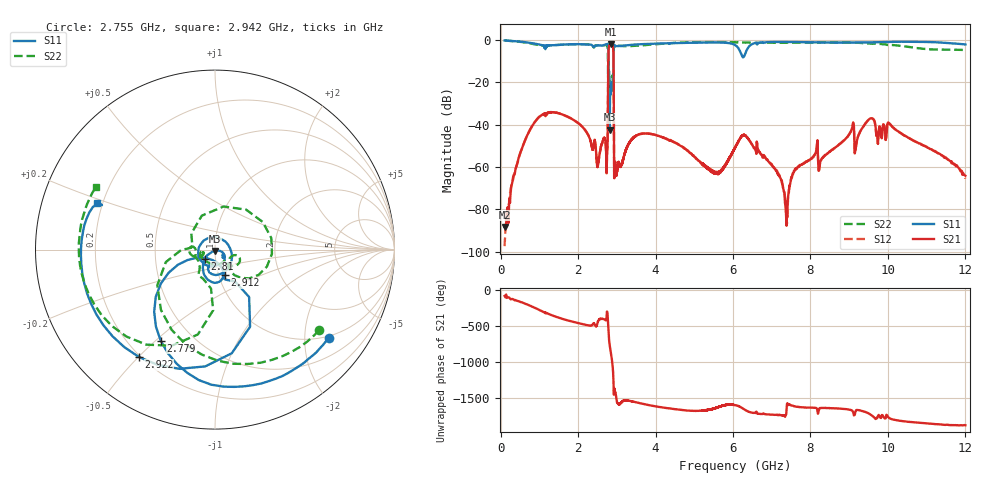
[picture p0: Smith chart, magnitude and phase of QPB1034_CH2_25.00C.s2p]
! TDS: k:\Engsetup\Winsaw\QPB1034_ALL
! Channel 1
! Ports=1 2
! seg 1=100.000000 1100.000000 51
! seg 2=1101.000000 1301.000000 201
! seg 3=1302.000000 2302.000000 101
! seg 4=2303.000000 3503.000000 1201
! seg 5=3504.000000 5204.000000 171
! seg 6=5205.000000 6405.000000 1201
! seg 7=6406.000000 8506.000000 211
! seg 8=8507.000000 12007.000000 176
! Points=3313
! FailCode=0
! Topology=ALL_SE(12)
!VNA Cal loaded =QPB1034_ALL_25C
!PS1(V)= 5.000
!PS(mA)= 0.427
!PS2(V)= 0.630
!PS(mA)= -0.002
!PS3(V)= 1.170
!PS(mA)= 0.000
!PS4(V)= 0.630
!PS(mA)= -0.002
!Temp (C)= 25.00
# MHz S DB R 50
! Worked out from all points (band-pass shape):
!   3313 points, 100 MHz to 12.01 GHz, reference 50 ohm
!   highest |S21| = -2.19 dB at 2.84 GHz (marker M1); lowest = -88.3 dB at 100 MHz (marker M2)
!   |S21| within 3 dB of the highest: 2.785 GHz to 2.911 GHz (126 MHz wide, 4.42 % of centre)
!   lowest |S11| = -42.4 dB at 2.817 GHz (marker M3), VSWR 1.02, Z = 50.1 - j0.758 ohm
!   |S11| at or under -10 dB: 2.784 GHz to 2.916 GHz (132.4 MHz wide, 4.65 % of centre)
!   |S22| runs from -23.7 to -0.3 dB; largest |S21 - S12| = 0.0046
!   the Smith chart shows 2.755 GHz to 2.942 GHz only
!   S11 on the Smith chart (normalised r, x): 2.755 GHz: 0.93, -2.61; 2.779 GHz: 0.33, -0.52; 2.81 GHz: 0.89, -0.09; 2.912 GHz: 1.07, -0.31; 2.922 GHz: 0.19, -0.50; 2.942 GHz: 0.18, +0.18
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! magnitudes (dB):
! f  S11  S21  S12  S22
! 100 MHz  -0.3  -88.3  -97.3  -0.3
! 240 MHz  -0.5  -76.9  -72.1  -0.5
! 500 MHz  -0.9  -53.6  -53.6  -0.9
! 1.1 GHz  -2.6  -35.1  -35.2  -2.8
! 2.434 GHz  -2.8  -47.7  -47.8  -2.8
! 2.502 GHz  -2.6  -60.0  -59.7  -2.6
! 2.738 GHz  -2.0  -61.4  -61.6  -2.4
! 2.755 GHz  -1.9  -51.0  -50.9  -2.7
! 2.779 GHz  -4.6  -10.7  -10.7  -10.3
! 2.81 GHz  -22.6  -2.5  -2.5  -19.9
! 2.817 GHz  -42.4  -2.4  -2.4  -21.8
! 2.84 GHz  -25.6  -2.2  -2.2  -21.7
! 2.899 GHz  -18.2  -3.4  -3.4  -19.4
! 2.912 GHz  -16.3  -5.5  -5.5  -15.7
! 2.922 GHz  -2.7  -38.4  -38.4  -2.7
! 2.942 GHz  -3.1  -58.8  -58.9  -2.5
! 3.744 GHz  -2.0  -44.2  -44.2  -2.5
! 5.406 GHz  -1.2  -61.0  -61.2  -1.1
! 6.295 GHz  -7.6  -44.9  -44.9  -1.2
! 7.376 GHz  -1.0  -84.4  -84.1  -1.4
! 9.747 GHz  -1.1  -49.1  -49.0  -1.9
! 12.01 GHz  -2.2  -64.1  -65.5  -4.8
